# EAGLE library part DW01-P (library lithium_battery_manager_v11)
One Cell Lithium-ion/Polymer Battery Protection IC The DW01-P battery protection IC is designed to protect lithium-ion/polymer battery from damage or degrading the lifetime due to overcharge, overdischarge, and/or overcurrent for one-cell lithium-ion/polymer battery powered systems, such as cellular phones. The ultra-small package and less required external components make it ideal to integrate the DW01-P into the limited space of battery pack. The accurate ±50mV overcharging detection voltage ensures safe and full utilization charging. The very low standby current drains little current from the cell while in storage.
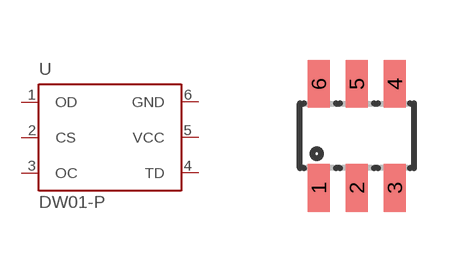
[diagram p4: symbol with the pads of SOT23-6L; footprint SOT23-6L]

Designator prefix -

## DW01-P  [SOT23-6L]
1  OD  pwr
2  CS  in
3  OC  pwr
4  TD  out
5  VCC  in
6  GND  out

## Footprint SOT23-6L (pad centres in mm)
Small Outline Transistor
smd 0.55 x 1.2: 1 -0.95,-1.3; 2 0,-1.3; 3 0.95,-1.3; 4 0.95,1.3; 5 0,1.3; 6 -0.95,1.3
